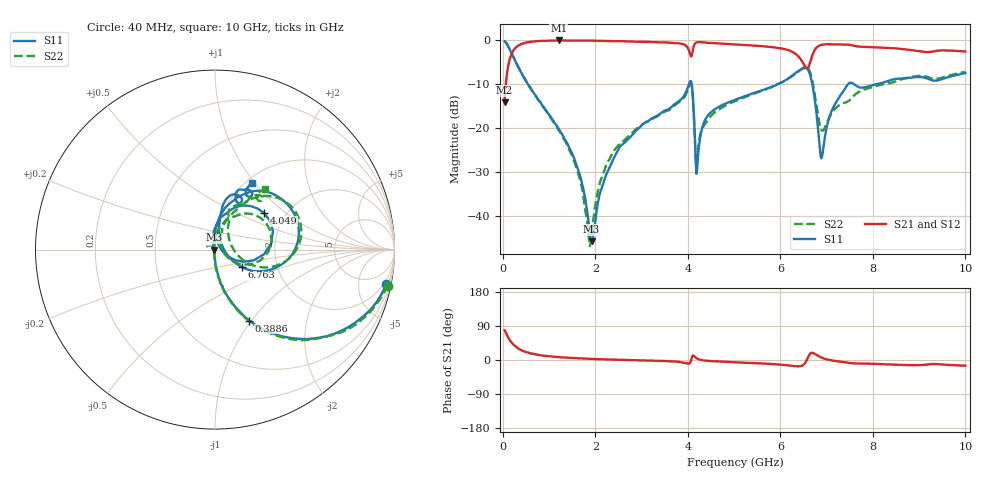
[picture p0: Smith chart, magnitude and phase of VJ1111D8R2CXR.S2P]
! VJ1111D8R2CXR
! DATE 03/04/2022  14:22
! CAPACITORS MOUNTED IN SERIES ON 25 MIL THICK MICROSTRIP SUBSTRATE
# GHz  S  MA  R  50.00
!  FREQ  S11M  S11A  S21M  S21A  S12M  S12A  S22M  S22A
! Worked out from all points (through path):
!   801 points, 40 MHz to 10 GHz, reference 50 ohm
!   highest |S21| = -0.01 dB at 1.21 GHz (marker M1); lowest = -14.1 dB at 40 MHz (marker M2)
!   group delay of S21, straight-line fit = 8.92 ps
!   lowest |S11| = -45.8 dB at 1.92 GHz (marker M3), VSWR 1.01, Z = 49.5 + j0.0133 ohm
!   |S11| at or under -10 dB: 546.9 MHz to 4.024 GHz (3.477 GHz wide, 152 % of centre); 4.086 GHz to 5.945 GHz (1.859 GHz wide, 37.1 % of centre); 6.691 GHz to 7.462 GHz (770.4 MHz wide, 10.9 % of centre)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
!   |S22| runs from -46.9 to -0.1 dB; largest |S21 - S12| = 0.011
!   S11 on the Smith chart (normalised r, x): 40 MHz: 1.33, -9.82; 388.6 MHz: 0.99, -0.97; 4.049 GHz: 1.54, +0.72; 6.763 GHz: 1.32, -0.27; 10 GHz: 1.06, +0.96
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0.04  0.9735 -11.4  0.1978 78.4  0.1991 78.5  0.983 -11.8
0.17695  0.7398 -42.0  0.6727 48.3  0.6723 48.6  0.7444 -42.1
0.3886  0.439 -64.3  0.9043 26.7  0.9082 26.6  0.4414 -64.5
1.2103  0.09739 -86.3  0.9994 7.5  1.003 7.4  0.09452 -87.7
1.7083  0.02387 -97.7  0.9976 4.0  1.003 3.9  0.02105 -101.7
1.91995  0.005132 178.5  0.9947 2.9  0.9984 2.8  0.006292 133.1
2.09425  0.01756 109.3  0.9908 2.1  0.9946 2.0  0.02332 99.2
2.3806  0.04327 103.9  0.981 1.1  0.9855 0.9  0.05271 89.6
3.36415  0.1413 85.7  0.9509 -2.3  0.9557 -2.4  0.1386 75.7
4.0489  0.3404 37.1  0.7035 -7.2  0.7069 -7.3  0.321 27.8
4.21075  0.04071 66.8  0.9553 3.3  0.9585 3.2  0.05053 52.5
4.4224  0.1371 86.4  0.9405 -2.2  0.9451 -2.3  0.1221 71.0
5.02  0.2102 79.0  0.903 -6.0  0.9068 -6.2  0.203 66.2
6.3397  0.4294 49.0  0.6975 -16.6  0.7005 -16.7  0.4223 45.0
6.5638  0.4808 14.3  0.4831 -1.9  0.4846 -2.0  0.4971 16.4
6.6883  0.3227 -20.7  0.6669 19.0  0.6699 18.8  0.3523 -14.8
6.763  0.1789 -33.1  0.806 14.9  0.8102 14.7  0.2114 -22.7
6.89995  0.04704 35.7  0.8938 5.9  0.8965 5.8  0.09394 17.8
7.09915  0.1522 80.8  0.9053 -0.8  0.9085 -0.9  0.1447 59.9
7.4602  0.3155 73.7  0.8965 -7.1  0.8996 -7.2  0.202 67.5
8.34415  0.347 69.3  0.8229 -11.8  0.8266 -11.9  0.3253 56.4
10  0.425 61.4  0.7464 -15.1  0.7495 -15.3  0.4375 50.2
